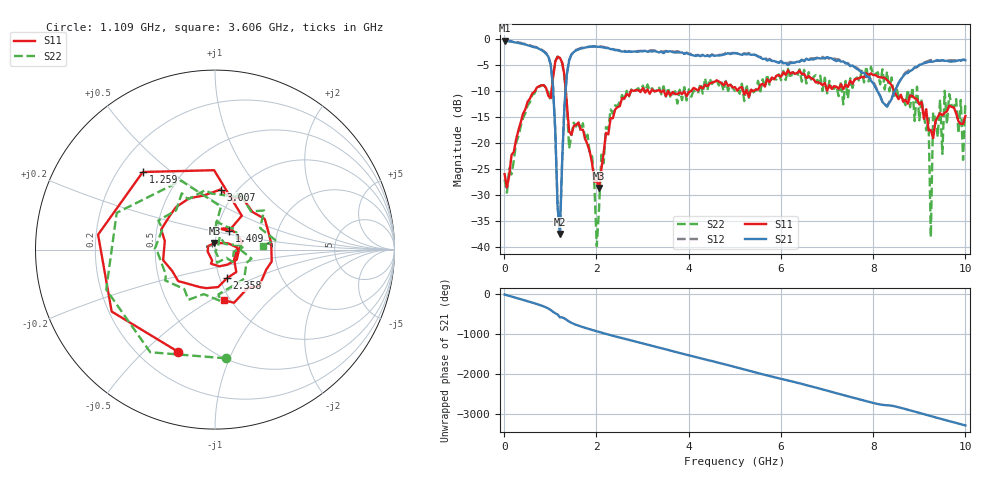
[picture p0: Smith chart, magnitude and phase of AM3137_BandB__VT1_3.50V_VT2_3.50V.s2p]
! Date/Time: Tue, Nov 13, 2018 4:52 PM
! Network Analyzer: Agilent Technologies E8364B Rev: A.07.50.67
! Sweep from 0.010 to 10.000 GHz, 201 Points, Sweep Type: LIN
! Power Supply: 3.501 V, 0.000 A
# Hz S DB R 50
!freq MagS11 AngS11 MagS21 AngS21 MagS12 AngS12 MagS22 AngS22
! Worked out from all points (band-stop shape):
!   201 points, 10 MHz to 10 GHz, reference 50 ohm
!   highest |S21| = -0.34 dB at 10 MHz (marker M1); lowest = -37.6 dB at 1.209 GHz (marker M2)
!   |S21| within 3 dB of the highest: 1.446 GHz to 4.436 GHz (2.989 GHz wide, 102 % of centre); 4.464 GHz to 5.498 GHz (1.033 GHz wide, 20.7 % of centre)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
!   lowest |S11| = -28.7 dB at 2.058 GHz (marker M3), VSWR 1.08, Z = 49.6 + j3.63 ohm
!   |S11| at or under -10 dB: start of sweep to 668.8 MHz; 1.336 GHz to 2.752 GHz (1.416 GHz wide, 69.3 % of centre); 8.452 GHz to end of sweep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
!   |S22| runs from -39.9 to -3.4 dB; largest |S21 - S12| = 0.03
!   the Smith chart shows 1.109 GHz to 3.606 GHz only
!   S11 on the Smith chart (normalised r, x): 1.109 GHz: 0.36, -0.64; 1.259 GHz: 0.30, +0.40; 1.409 GHz: 1.14, +0.24; 2.358 GHz: 1.08, -0.35; 3.007 GHz: 0.84, +0.64; 3.606 GHz: 0.93, -0.57
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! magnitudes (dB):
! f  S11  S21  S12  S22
! 10 MHz  -26.0  -0.3  -0.3  -27.0
! 959 MHz  -11.0  -3.4  -3.4  -10.3
! 1.109 GHz  -4.4  -17.8  -17.7  -4.3
! 1.209 GHz  -3.7  -37.6  -37.6  -3.8
! 1.259 GHz  -4.6  -23.3  -23.2  -4.7
! 1.409 GHz  -17.8  -4.2  -4.1  -21.1
! 1.708 GHz  -17.5  -1.8  -1.7  -16.3
! 2.008 GHz  -27.4  -1.5  -1.4  -39.9
! 2.058 GHz  -28.7  -1.5  -1.4  -32.6
! 2.358 GHz  -15.3  -2.0  -2.0  -14.4
! 3.007 GHz  -9.5  -2.4  -2.3  -9.0
! 3.357 GHz  -9.8  -2.6  -2.4  -9.2
! 3.606 GHz  -10.9  -2.4  -2.4  -11.4
! 5.005 GHz  -9.3  -2.7  -2.7  -10.0
! 6.703 GHz  -7.7  -4.0  -3.8  -7.4
! 8.352 GHz  -8.4  -12.3  -12.1  -10.1
! 9.201 GHz  -17.6  -4.4  -4.2  -15.2
! 9.251 GHz  -17.5  -4.4  -4.1  -38.1
! 9.301 GHz  -19.1  -4.4  -4.2  -14.1
! 9.9 GHz  -16.4  -4.1  -4.2  -11.8
! 9.95 GHz  -16.3  -4.0  -4.0  -23.3
! 10 GHz  -14.8  -4.1  -4.0  -12.1
